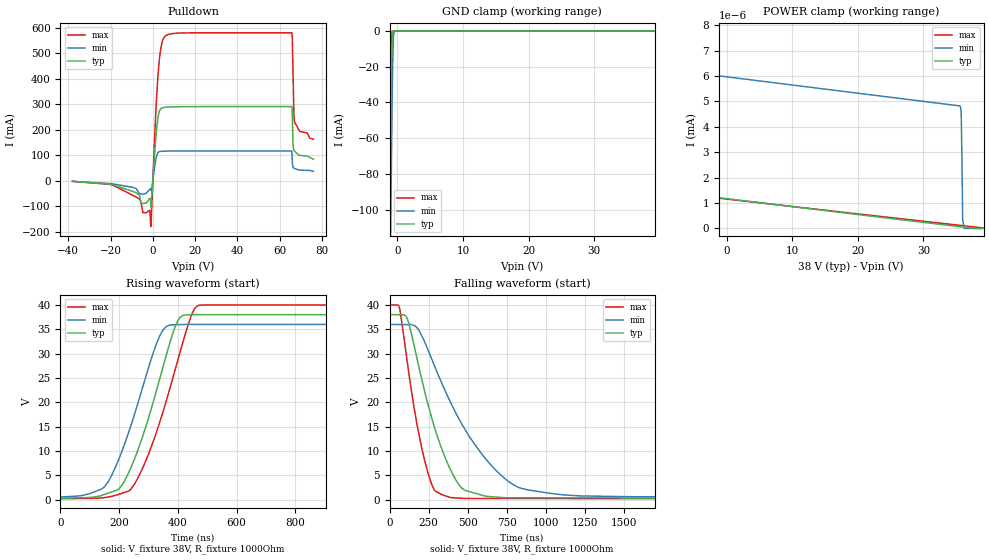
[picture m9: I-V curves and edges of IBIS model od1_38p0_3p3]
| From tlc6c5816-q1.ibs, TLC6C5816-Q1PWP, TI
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|   od1_38p0_3p3 Model
[Model]   od1_38p0_3p3
Model_type   Open_drain
Polarity   Inverting
Vmeas = 19
Vref = 38
Cref = 2pF
Rref = 1000
|   typ   min   max
C_comp   2.628pF   2.247pF   2.752pF
| Where Nom  PVT is Nominal Process, 38.0V, 27C
|   Fast PVT is Strong Process,  40.0V, -40C
|   Slow PVT is Weak Process,   36.0V, 150C
[Voltage Range]   38   36   40
|Junction Temperature
[Temperature Range]   27   150   -40
[Pullup Reference]   38   36   40
[Pulldown Reference]   0   -0   0
[Power Clamp Reference]   38   36   40
[GND Clamp Reference]   0   0   0
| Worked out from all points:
|   slope of the pulldown table from 0 to 5.7 V, typ, clamps not added: 19.8 ohm
|   GND clamp passes 1 mA (typ) near -0.73 V on its own axis
|   falling waveform, V_fixture 38V, R_fixture 1000Ohm: 20-80 % time 201ns typ, 366ns min, 127ns max; typ from 38 V to 0.29 V
|   rising waveform, V_fixture 38V, R_fixture 1000Ohm: 20-80 % time 115ns typ, 115ns min, 124ns max; typ from 0.29 V to 38 V
[Pulldown]
|   Voltage   I(typ)   I(min)   I(max)
-38V      -2.502mA   -2.646mA   -2.514mA
-7.904V   -46.82mA   -30.74mA   -64.06mA
-1.52V    -70.43mA   -34.72mA   -115.6mA
-950mV    -91.2mA    -31.51mA   -179.8mA
1.558V    181.3mA    88.13mA    291.7mA
3.04V     271.2mA    113.5mA    470.3mA
4.864V    286.2mA    115.5mA    554.4mA
8.056V    289mA      116mA      574.7mA
65.74V    290.3mA    115.2mA    579.4mA
66.31V    143.6mA    53.49mA    429.1mA
66.99V    116.6mA    48.24mA    230.9mA
76V       84.21mA    36.57mA    162.4mA
[GND Clamp]
|   Voltage   I(typ)   I(min)   I(max)
-38V      -18.95A    -18.51A    -19.22A
-1.292V   -161.2mA   -209.4mA   -136.1mA
-1.178V   -117.5mA   -166.8mA   -91.39mA
-1.064V   -75.38mA   -125.1mA   -48.96mA
-950mV    -36.53mA   -85.06mA   -13.12mA
-836mV    -7.654mA   -48.07mA   -310uA
-722mV    -266uA     -17.89mA   -2.372uA
-608mV    -5.048uA   -2.691mA   -37.32nA
-494mV    -96.2nA    -186.5uA   -1.113nA
-266mV    -44.51pA   -662nA     -4.297pA
76V       0A         0A         0A
[POWER Clamp]
|   Voltage   I(typ)   I(min)   I(max)
-38V      4.427A     3.422A     5.462A
-29.56V   655.6mA    11.74uA    1.527A
-28.77V   333.6mA    6.877nA    1.172A
-27.85V   4.302mA    6.854nA    781mA
-26.49V   1.98nA     6.818nA    220.5mA
-9.5V     1.468nA    6.276nA    1.433nA
35.53V    68.2pA     4.821nA    120.6pA
35.76V    61.3pA     4.592nA    114pA
35.87V    57.85pA    2.841nA    110.7pA
35.99V    54.41pA    348.9pA    107.5pA
36.21V    47.53pA    0A         100.9pA
76V       0A         0A         0A
[Ramp]
R_load = 1000
|   typ   min   max
dV/dt_r   22.6262/1.15342e-07   21.2728/1.15104e-07   23.8823/1.2374e-07
dV/dt_f   22.6262/2.01372e-07   21.2728/3.65319e-07   23.8823/1.26685e-07
[Falling Waveform]
V_fixture = 38V
V_fixture_min = 36V
V_fixture_max = 40V
R_fixture = 1000Ohm
C_fixture = 0F
|   Time   V(typ)   V(min)   V(max)
0s        38V        36V        40V
63.4ns    37.98V     35.98V     39.4V
113.3ns   37.23V     35.96V     28.36V
223.2ns   22.48V     32.53V     8.264V
280.4ns   15.65V     28.09V     2.392V
324.3ns   11.34V     24.7V      1.224V
464.6ns   2.313V     15.46V     283mV
659.5ns   588.3mV    6.77V      240.9mV
839.5ns   385.7mV    2.376V     236.5mV
2.5us     289.6mV    545.4mV    196.2mV
[Rising Waveform]
V_fixture = 38V
V_fixture_min = 36V
V_fixture_max = 40V
R_fixture = 1000Ohm
C_fixture = 0F
|   Time   V(typ)   V(min)   V(max)
0s        289.6mV    545.4mV    196.2mV
151.5ns   1.108V     2.743V     433mV
200.5ns   2.292V     8.586V     1.124V
247.9ns   7.723V     16.72V     2.809V
300.5ns   16.86V     27.22V     9.452V
347.4ns   26.85V     34.67V     17.7V
404.1ns   37.18V     35.95V     29.59V
446.6ns   37.98V     36V        37.94V
470.9ns   38V        36V        39.91V
2.5us     38V        36V        40V
